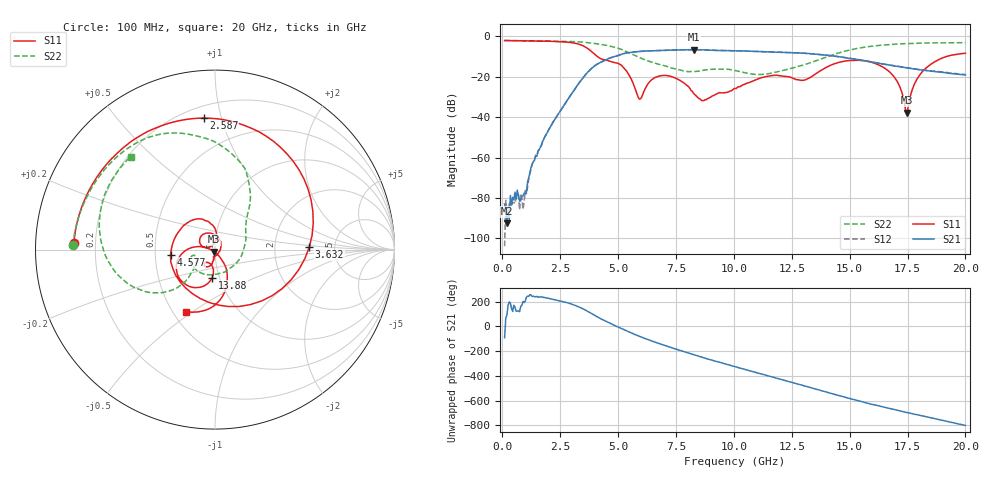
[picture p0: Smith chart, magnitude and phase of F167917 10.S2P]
!  2-Port S-parameters saved by WinCal
! VAR MeasName=S-Parameters (CALIBRATED_DATA) read from VNA (N5242A)
! VAR MeasDate=2016-11-22 9:00:11
! VAR NAME=F167917 10
! VAR FILENAME=F167917 10.S2P
! VAR DATE=2016-11-22 9:00:11
! VAR PHYS_PORTS=1,2
# Hz S DB R 50
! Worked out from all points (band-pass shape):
!   401 points, 100 MHz to 20 GHz, reference 50 ohm
!   highest |S21| = -6.55 dB at 8.259 GHz (marker M1); lowest = -92.6 dB at 199.5 MHz (marker M2)
!   |S21| within 3 dB of the highest: 4.987 GHz to 14.18 GHz (9.194 GHz wide, 95.9 % of centre)
!   lowest |S11| = -37.8 dB at 17.46 GHz (marker M3), VSWR 1.03, Z = 49.3 - j1.06 ohm
!   |S11| at or under -10 dB: 4.108 GHz to 19.17 GHz (15.07 GHz wide, 129 % of centre)
!   |S22| runs from -18.9 to -2.0 dB; largest |S21 - S12| = 0.0041
!   S11 on the Smith chart (normalised r, x): 100 MHz: 0.12, +0.02; 2.587 GHz: 0.28, +0.88; 3.632 GHz: 3.21, +0.11; 4.577 GHz: 0.60, -0.04; 13.88 GHz: 0.92, -0.30; 20 GHz: 0.58, -0.47
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1e8  -2.09 177.3  -83.09 -93.6  -103.91 -21.4  -2.03 178.3
1.995e8  -2.09 174.7  -92.64 90.1  -86.14 109.0  -2.04 176.7
9.4575e8  -2.21 154.7  -77.56 -168.1  -81.46 -145.9  -2.17 165.1
1.34375e9  -2.28 143.3  -61.95 -116.2  -61.98 -116.3  -2.23 158.9
2.5875e9  -2.67 94.9  -35.47 -159.0  -35.46 -159.7  -2.46 137.6
3.43325e9  -4.40 27.3  -21.27 145.5  -21.30 145.4  -2.83 118.9
3.63225e9  -5.59 1.4  -18.46 126.6  -18.46 126.6  -3.02 113.8
4.03025e9  -9.26 -67.1  -14.28 84.2  -14.23 84.3  -3.59 103.3
4.5775e9  -12.06 -173.3  -11.01 30.9  -10.97 30.6  -4.65 87.5
5.274e9  -15.90 103.1  -8.43 -29.2  -8.44 -29.4  -7.14 65.2
5.92075e9  -31.07 121.2  -7.48 -80.9  -7.47 -81.0  -10.45 50.6
6.7665e9  -19.71 145.1  -6.96 -138.9  -6.97 -139.1  -13.86 32.5
8.259e9  -28.19 31.3  -6.55 130.9  -6.57 131.0  -17.34 -70.7
1.005e10  -25.78 -99.8  -7.14 33.6  -7.14 33.7  -16.96 -161.8
1.19405e10  -19.44 -122.9  -7.87 -63.2  -7.82 -63.3  -17.33 -143.3
1.338325e10  -19.75 -96.3  -8.65 -138.9  -8.64 -138.6  -12.73 -133.1
1.388075e10  -16.06 -95.7  -9.19 -165.3  -9.15 -164.8  -10.67 -134.5
1.5423e10  -11.88 -141.7  -11.66 116.4  -11.58 116.2  -5.77 -157.5
1.67165e10  -17.54 175.5  -14.17 56.6  -14.20 57.0  -4.06 178.9
1.746275e10  -37.79 -123.7  -15.61 24.3  -15.49 25.1  -3.58 166.8
1.825875e10  -16.10 -64.1  -16.84 -8.2  -16.73 -7.9  -3.29 154.9
2e10  -8.37 -115.3  -19.12 -80.7  -18.90 -81.0  -3.12 132.1
